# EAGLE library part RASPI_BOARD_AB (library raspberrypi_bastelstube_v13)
Raspberry Pi GPIO connector with markings for the outer dimensions of the Raspberry Pi board model A or B with different sets of drill holes or mounting pads for model B Revision 2.0
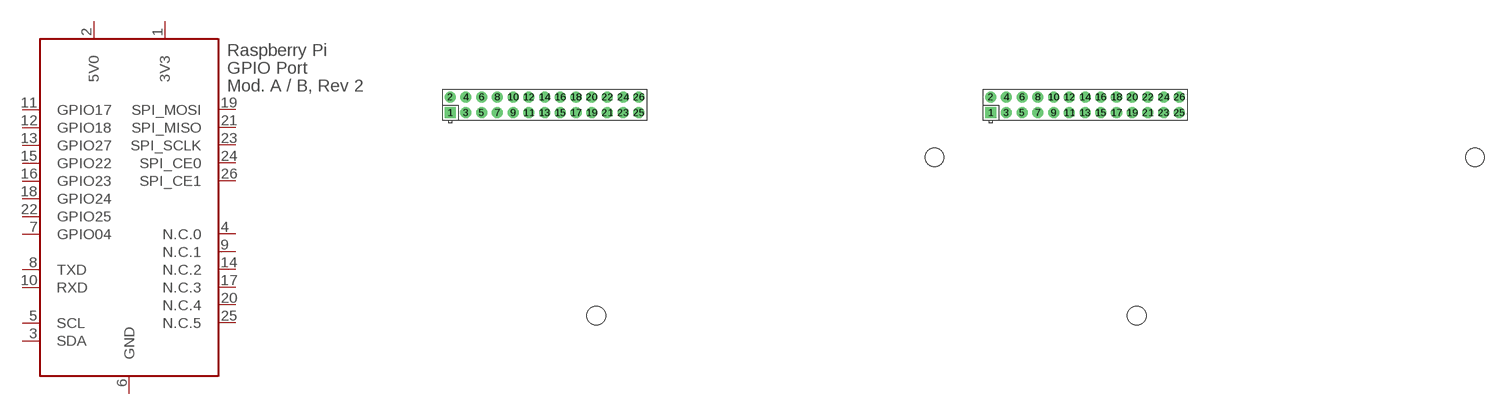
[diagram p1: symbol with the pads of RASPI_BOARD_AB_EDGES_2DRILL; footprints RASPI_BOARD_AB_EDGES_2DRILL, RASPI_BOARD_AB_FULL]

Designator prefix X

## RASPI_BOARD_AB_E2  [RASPI_BOARD_AB_EDGES_2DRILL]
1  3V3  pwr
2  5V0  pwr
3  SDA
4  N.C.0  nc
5  SCL
6  GND  pwr
7  GPIO04
8  TXD
9  N.C.1  nc
10  RXD
11  GPIO17
12  GPIO18
13  GPIO27
14  N.C.2  nc
15  GPIO22
16  GPIO23
17  N.C.3  nc
18  GPIO24
19  SPI_MOSI
20  N.C.4  nc
21  SPI_MISO
22  GPIO25
23  SPI_SCLK
24  SPI_CE0
25  N.C.5  nc
26  SPI_CE1

## RASPI_BOARD_AB_F  [RASPI_BOARD_AB_FULL]
Pads as for RASPI_BOARD_AB_EDGES_2DRILL

## RASPI_BOARD_AB_E1  [RASPI_BOARD_AB_EDGES_1DRILL]
Pads as for RASPI_BOARD_AB_EDGES_2DRILL

## RASPI_BOARD_AB_TD  [RASPI_BOARD_AB_THIN_DRILL]
Pads as for RASPI_BOARD_AB_EDGES_2DRILL

## RASPI_BOARD_AB_E1P  [RASPI_BOARD_AB_EDGES_1DRILL_PAD]
Pads as for RASPI_BOARD_AB_EDGES_2DRILL

## RASPI_BOARD_AB_E2P  [RASPI_BOARD_AB_EDGES_2DRILL_PAD]
Pads as for RASPI_BOARD_AB_EDGES_2DRILL

## RASPI_BOARD_AB_FP  [RASPI_BOARD_AB_FULL_PAD]
Pads as for RASPI_BOARD_AB_EDGES_2DRILL

## RASPI_BOARD_AB_TP  [RASPI_BOARD_AB_THIN_PAD]
Pads as for RASPI_BOARD_AB_EDGES_2DRILL

## RASPI_BOARD_AB_TB  [RASPI_BOARD_AB_THIN_BOT]
Pads as for RASPI_BOARD_AB_EDGES_2DRILL

## RASPI_BOARD_AB_E0  [RASPI_BOARD_AB_EDGES_0DRILL]
Pads as for RASPI_BOARD_AB_EDGES_2DRILL

## RASPI_BOARD_AB_T  [RASPI_BOARD_AB_THIN]
Pads as for RASPI_BOARD_AB_EDGES_2DRILL

## Footprint RASPI_BOARD_AB_EDGES_2DRILL (pad centres in mm)
Raspberry Pi board model A / B, outline is only marked by its edges including 2 drill holes for Model B Revision 2.0
drill 1 pad 1.778 square: 1 1.905,50.8
drill 1 pad 1.778: 2 1.905,53.34; 3 4.445,50.8; 4 4.445,53.34; 5 6.985,50.8; 6 6.985,53.34; 7 9.525,50.8; 8 9.525,53.34; 9 12.065,50.8; 10 12.065,53.34; 11 14.605,50.8; 12 14.605,53.34; 13 17.145,50.8; 14 17.145,53.34; 15 19.685,50.8; 16 19.685,53.34; 17 22.225,50.8; 18 22.225,53.34; 19 24.765,50.8; 20 24.765,53.34; 21 27.305,50.8; 22 27.305,53.34; 23 29.845,50.8; 24 29.845,53.34; 25 32.385,50.8; 26 32.385,53.34
hole 3 at 25.5,18
hole 3 at 80.1,43.6

## Footprint RASPI_BOARD_AB_FULL (pad centres in mm)
Raspberry Pi board, full outline with position of big connectors + components including drill holes for Model B Revision 2.0
drill 1 pad 1.778 square: 1 1.905,50.8
drill 1 pad 1.778: 2 1.905,53.34; 3 4.445,50.8; 4 4.445,53.34; 5 6.985,50.8; 6 6.985,53.34; 7 9.525,50.8; 8 9.525,53.34; 9 12.065,50.8; 10 12.065,53.34; 11 14.605,50.8; 12 14.605,53.34; 13 17.145,50.8; 14 17.145,53.34; 15 19.685,50.8; 16 19.685,53.34; 17 22.225,50.8; 18 22.225,53.34; 19 24.765,50.8; 20 24.765,53.34; 21 27.305,50.8; 22 27.305,53.34; 23 29.845,50.8; 24 29.845,53.34; 25 32.385,50.8; 26 32.385,53.34
hole 3 at 25.5,18
hole 3 at 80.1,43.6

## Footprint RASPI_BOARD_AB_EDGES_1DRILL (pad centres in mm)
Raspberry Pi board model A / B, outline is only marked by its edges including 1 drill hole for Model B Revision 2.0
drill 1 pad 1.778 square: 1 1.905,50.8
drill 1 pad 1.778: 2 1.905,53.34; 3 4.445,50.8; 4 4.445,53.34; 5 6.985,50.8; 6 6.985,53.34; 7 9.525,50.8; 8 9.525,53.34; 9 12.065,50.8; 10 12.065,53.34; 11 14.605,50.8; 12 14.605,53.34; 13 17.145,50.8; 14 17.145,53.34; 15 19.685,50.8; 16 19.685,53.34; 17 22.225,50.8; 18 22.225,53.34; 19 24.765,50.8; 20 24.765,53.34; 21 27.305,50.8; 22 27.305,53.34; 23 29.845,50.8; 24 29.845,53.34; 25 32.385,50.8; 26 32.385,53.34
hole 3 at 80.1,43.6

## Footprint RASPI_BOARD_AB_THIN_DRILL (pad centres in mm)
Raspberry Pi board - Thin version with only the width of the GPIO connector and 1 drill hole
drill 1 pad 1.778 square: 1 1.905,50.8
drill 1 pad 1.778: 2 1.905,53.34; 3 4.445,50.8; 4 4.445,53.34; 5 6.985,50.8; 6 6.985,53.34; 7 9.525,50.8; 8 9.525,53.34; 9 12.065,50.8; 10 12.065,53.34; 11 14.605,50.8; 12 14.605,53.34; 13 17.145,50.8; 14 17.145,53.34; 15 19.685,50.8; 16 19.685,53.34; 17 22.225,50.8; 18 22.225,53.34; 19 24.765,50.8; 20 24.765,53.34; 21 27.305,50.8; 22 27.305,53.34; 23 29.845,50.8; 24 29.845,53.34; 25 32.385,50.8; 26 32.385,53.34
hole 3 at 25.5,18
